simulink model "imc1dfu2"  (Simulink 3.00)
settings: Solver=ode45  SolverMode=SingleTasking  StartTime=0.0  StopTime=50  MaxStep=st_size  RelTol=1e-5  AbsTol=1e-6
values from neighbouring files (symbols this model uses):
  Disturb = Setpoint    [mimo_MSF1DF_sim.m]    (also in mimo_MSF2DF_sim.m)
  Satlb = temp1    [cback.m]    (also in imcmenu.m = str2num(satlbs))
  Satub = temp1    [cback.m]    (also in imcmenu.m = str2num(satubs))
  Setpoint = zeros(1,n)    [mimo_MSF1DF_sim.m]    (also in mimo_MSF2DF_sim.m)
undefined symbols (not defined in the file or in its folder): Csden, Csnum, pdeadx, XdenPs, XnumPs

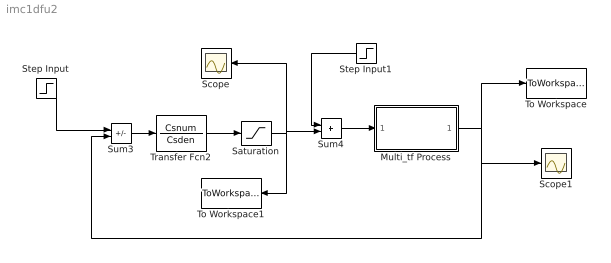
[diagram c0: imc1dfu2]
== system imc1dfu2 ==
  Multi_tf Process : Subsystem
  Saturation : Saturate  UpperLimit=Satub  LowerLimit=Satlb
  Scope : Scope
  Scope1 : Scope
  Step Input : Step  Time=0  Before=0  After=Setpoint  SampleTime=0
  Step Input1 : Step  Orientation=left  Time=0  Before=0  After=Disturb  SampleTime=0
  Sum3 : Sum  Inputs=+-  SaturateOnIntegerOverflow=on
  Sum4 : Sum  Inputs=++  SaturateOnIntegerOverflow=on
  To Workspace : ToWorkspace  VariableName=simout  SampleTime=-1  SaveFormat=Matrix
  To Workspace1 : ToWorkspace  VariableName=effort  SampleTime=-1  SaveFormat=Matrix
  Transfer Fcn2 : TransferFcn  Numerator=Csnum  Denominator=Csden
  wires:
  Sum3/1 -> Transfer Fcn2/1
  Transfer Fcn2/1 -> Saturation/1
  Step Input/1 -> Sum3/1
  Step Input1/1 -> Sum4/1
  Saturation/1 -> Sum4/2, To Workspace1/1, Scope/1
  Sum4/1 -> Multi_tf Process/1(In1)
  Multi_tf Process/1(Out1) -> Sum3/2, To Workspace/1, Scope1/1

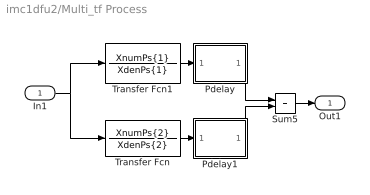
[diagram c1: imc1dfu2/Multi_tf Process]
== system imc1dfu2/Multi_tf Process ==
  In1 : Inport  Port=1  PortWidth=-1  SampleTime=-1  DataType=auto
  Pdelay : Subsystem
  Pdelay1 : Subsystem
  Sum5 : Sum  Inputs=++  SaturateOnIntegerOverflow=on
  Transfer Fcn : TransferFcn  Numerator=XnumPs{2}  Denominator=XdenPs{2}
  Transfer Fcn1 : TransferFcn  Numerator=XnumPs{1}  Denominator=XdenPs{1}
  Out1 : Outport  Port=1  InitialOutput=0
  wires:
  Transfer Fcn1/1 -> Pdelay/1(In1)
  Transfer Fcn/1 -> Pdelay1/1(In1)
  In1/1 -> Transfer Fcn1/1, Transfer Fcn/1
  Sum5/1 -> Out1/1
  Pdelay/1(Out1) -> Sum5/1
  Pdelay1/1(Out1) -> Sum5/2

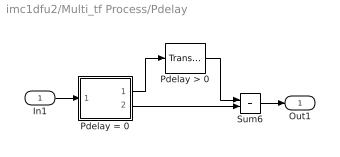
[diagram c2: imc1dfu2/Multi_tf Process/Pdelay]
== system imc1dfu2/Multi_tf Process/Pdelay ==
  In1 : Inport  Port=1  PortWidth=-1  SampleTime=-1  DataType=auto
  Pdelay > 0 : TransportDelay  DelayTime=pdeadx(1)  InitialInput=0  BufferSize=1024
  Pdelay = 0 : Subsystem  Description=pass input signal through out1 if condition is true.
  Sum6 : Sum  Inputs=++  SaturateOnIntegerOverflow=on
  Out1 : Outport  Port=1
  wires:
  Pdelay = 0/1(Out2) -> Pdelay > 0/1
  Pdelay > 0/1 -> Sum6/1
  Pdelay = 0/2(Out1) -> Sum6/2
  In1/1 -> Pdelay = 0/1(In)
  Sum6/1 -> Out1/1

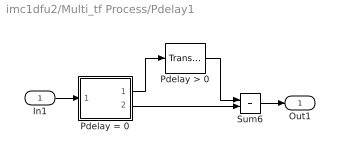
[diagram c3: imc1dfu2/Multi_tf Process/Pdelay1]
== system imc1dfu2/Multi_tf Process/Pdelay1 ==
  In1 : Inport  Port=1  PortWidth=-1  SampleTime=-1  DataType=auto
  Pdelay > 0 : TransportDelay  DelayTime=pdeadx(2)  InitialInput=0  BufferSize=1024
  Pdelay = 0 : Subsystem  Description=pass input signal through out1 if condition is true.
  Sum6 : Sum  Inputs=++  SaturateOnIntegerOverflow=on
  Out1 : Outport  Port=1
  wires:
  Pdelay = 0/1(Out2) -> Pdelay > 0/1
  Pdelay > 0/1 -> Sum6/1
  Pdelay = 0/2(Out1) -> Sum6/2
  In1/1 -> Pdelay = 0/1(In)
  Sum6/1 -> Out1/1

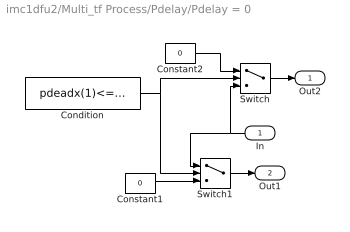
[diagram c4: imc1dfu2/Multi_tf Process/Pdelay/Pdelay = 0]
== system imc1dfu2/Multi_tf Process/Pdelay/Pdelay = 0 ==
  In : Inport  Orientation=left  Port=1  PortWidth=-1  SampleTime=-1  DataType=auto
  Condition : Constant  Value=pdeadx(1)<=3*eps
  Constant1 : Constant  Value=0
  Constant2 : Constant  Value=0
  Switch : Switch  Threshold=1
  Switch1 : Switch  Threshold=1
  Out2 : Outport  Port=1  InitialOutput=0
  Out1 : Outport  Port=2  InitialOutput=0
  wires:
  In/1 -> Switch/3, Switch1/1
  Condition/1 -> Switch1/2, Switch/2
  Constant1/1 -> Switch1/3
  Constant2/1 -> Switch/1
  Switch/1 -> Out2/1
  Switch1/1 -> Out1/1

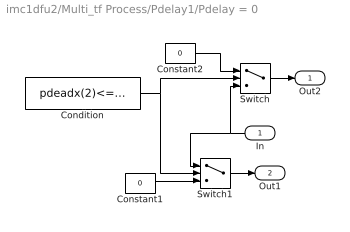
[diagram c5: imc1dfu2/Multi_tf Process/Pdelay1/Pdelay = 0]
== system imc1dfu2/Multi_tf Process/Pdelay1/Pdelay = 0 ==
  In : Inport  Orientation=left  Port=1  PortWidth=-1  SampleTime=-1  DataType=auto
  Condition : Constant  Value=pdeadx(2)<=3*eps
  Constant1 : Constant  Value=0
  Constant2 : Constant  Value=0
  Switch : Switch  Threshold=1
  Switch1 : Switch  Threshold=1
  Out2 : Outport  Port=1  InitialOutput=0
  Out1 : Outport  Port=2  InitialOutput=0
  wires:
  In/1 -> Switch/3, Switch1/1
  Condition/1 -> Switch1/2, Switch/2
  Constant1/1 -> Switch1/3
  Constant2/1 -> Switch/1
  Switch/1 -> Out2/1
  Switch1/1 -> Out1/1
